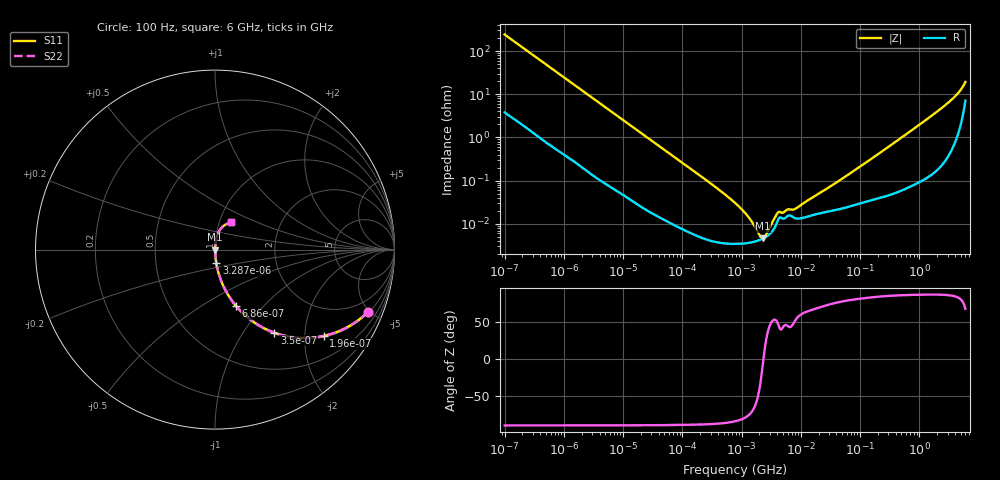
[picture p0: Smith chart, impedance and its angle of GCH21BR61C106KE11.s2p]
!Murata Part Number: GCH21BR61C106KE11
!These Parameters are Measured in Series Mode Connection
!Data Generated on Jun 19, 2026
!  o--ll--o
!Port1  Port2
!  o------o
!Operation Temp=25[degC], DC Bias Voltage=0[V]
!Freq. Start=100[Hz] Stop=6[GHz] 401[Steps]
# Hz S RI R 50
!Freq.(Hz) S11(Real) S11(Imag) S21(Real) S21(Imag) S12(Real) S12(Imag) S22(Real) S22(Imag)
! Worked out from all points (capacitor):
!   401 points, 100 Hz to 6 GHz, reference 50 ohm
!   read as one part in series: C = 6.57 uF near 109 Hz
!   lowest |Z| = 4.59 mohm at 2.269 MHz (marker M1)
!   series resonance near 2.335 MHz, so ESL is about 710 pH
!   S11 on the Smith chart (normalised r, x): 100 Hz: 1.08, -4.83; 196 Hz: 1.04, -2.49; 350 Hz: 1.02, -1.40; 686 Hz: 1.01, -0.72; 3.287 kHz: 1.00, -0.15; 6 GHz: 1.14, +0.36
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100  0.8499 -0.3494  0.1501 0.3494  0.1501 0.3494  0.8499 -0.3494
137  0.7549 -0.4223  0.2451 0.4223  0.2451 0.4223  0.7549 -0.4223
196  0.6053 -0.4808  0.3947 0.4808  0.3947 0.4808  0.6053 -0.4808
350  0.3305 -0.4626  0.6695 0.4626  0.6695 0.4626  0.3305 -0.4626
686  0.1181 -0.3149  0.8819 0.3149  0.8819 0.3149  0.1181 -0.3149
1073  0.0537 -0.2173  0.9463 0.2173  0.9463 0.2173  0.0537 -0.2173
2008  0.0171 -0.1217  0.9829 0.1217  0.9829 0.1217  0.0171 -0.1217
3287  0.00698 -0.0755  0.993 0.0755  0.993 0.0755  0.00698 -0.0755
40335  0.000184 -0.00637  0.9998 0.00637  0.9998 0.00637  0.000184 -0.00637
316350  4.04e-05 -0.000817  1 0.000817  1 0.000817  4.04e-05 -0.000817
774597  3.44e-05 -0.000304  1 0.000304  1 0.000304  3.44e-05 -0.000304
1585629  3.82e-05 -9.05e-05  1 9.05e-05  1 9.05e-05  3.82e-05 -9.05e-05
2268635  4.54e-05 -6.6e-06  1 6.6e-06  1 6.6e-06  4.54e-05 -6.6e-06
3103719  6.12e-05 6.9e-05  0.9999 -6.9e-05  0.9999 -6.9e-05  6.12e-05 6.9e-05
4246196  0.000133 0.000134  0.9999 -0.000134  0.9999 -0.000134  0.000133 0.000134
7947587  0.000136 0.000173  0.9999 -0.000173  0.9999 -0.000173  0.000136 0.000173
1.555665e7  0.000158 0.000372  0.9998 -0.000372  0.9998 -0.000372  0.000158 0.000372
4.764863e7  0.000224 0.00104  0.9998 -0.00104  0.9998 -0.00104  0.000224 0.00104
3.124326e8  0.0005 0.00624  0.9995 -0.00624  0.9995 -0.00624  0.0005 0.00624
2.679998e9  0.00567 0.054  0.9943 -0.054  0.9943 -0.054  0.00567 0.054
4.193612e9  0.0175 0.092  0.9825 -0.092  0.9825 -0.092  0.0175 0.092
6e9  0.0915 0.1513  0.9085 -0.1513  0.9085 -0.1513  0.0915 0.1513
